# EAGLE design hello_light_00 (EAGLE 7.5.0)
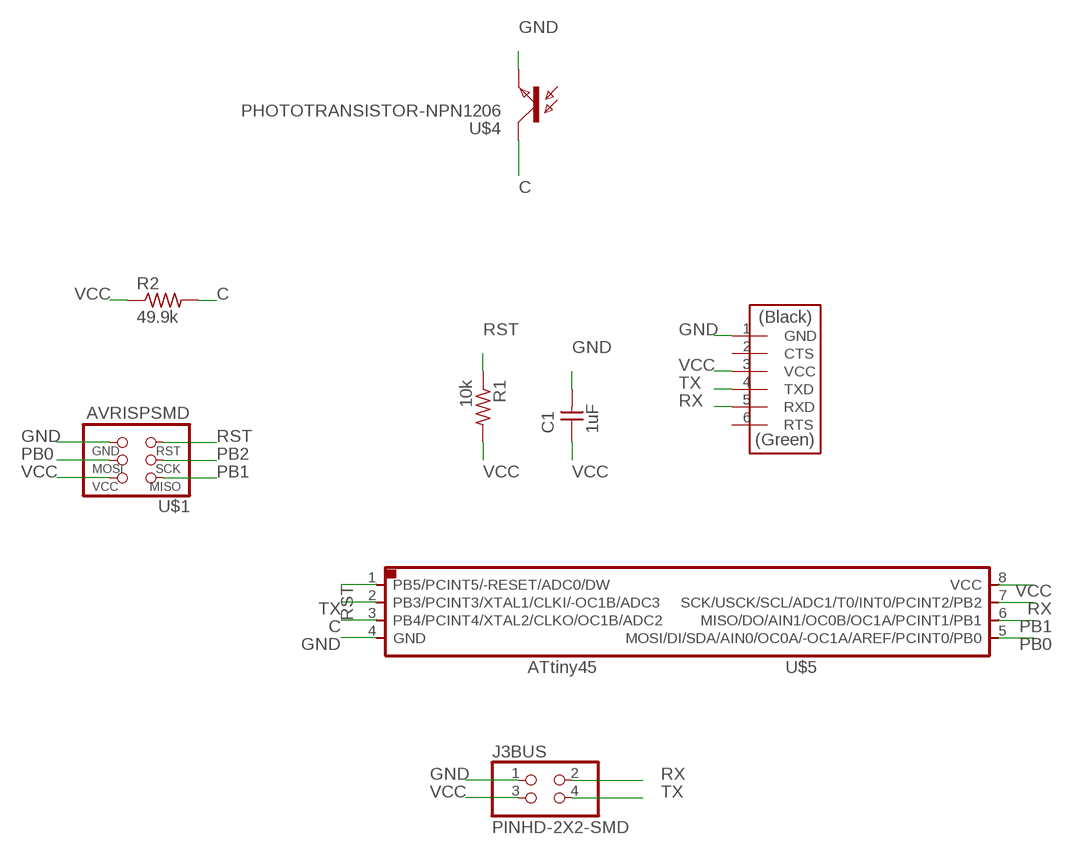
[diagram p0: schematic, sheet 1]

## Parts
C1  1uF  CAP-UNPOLARIZEDFAB  [C1206FAB]
J2FTDI  FTDI-SMD-HEADER  [1X06SMD]
J3BUS  PINHD-2X2-SMD  [2X02SMD]
R1  10k  RES-US1206FAB  [R1206FAB]
R2  49.9k  RES-US1206FAB  [R1206FAB]
U$1  AVRISPSMD  [2X03SMD]
U$4  PHOTOTRANSISTOR-NPN1206  [OP1206]
U$5  ATTINY45SI  [SOIC8]

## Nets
C: R2.2 U$4.COLLECTOR(C) U$5.3(PB4/PCINT4/XTAL2/CLKO/OC1B/ADC2)
GND: C1.2 J2FTDI.1(GND) J3BUS.1 U$1.6(GND) U$4.EMITTER(E) U$5.4(GND)
PB0: U$1.4(MOSI) U$5.5(MOSI/DI/SDA/AIN0/OC0A/-OC1A/AREF/PCINT0/PB0)
PB1: U$1.1(MISO) U$5.6(MISO/DO/AIN1/OC0B/OC1A/PCINT1/PB1)
PB2: U$1.3(SCK)
RST: R1.1 U$1.5(RST) U$5.1(PB5/PCINT5/-RESET/ADC0/DW)
RX: J2FTDI.5(RXD) J3BUS.2 U$5.7(SCK/USCK/SCL/ADC1/T0/INT0/PCINT2/PB2)
TX: J2FTDI.4(TXD) J3BUS.4 U$5.2(PB3/PCINT3/XTAL1/CLKI/-OC1B/ADC3)
VCC: C1.1 J2FTDI.3(VCC) J3BUS.3 R1.2 R2.1 U$1.2(VCC) U$5.8(VCC)
Unconnected: J2FTDI.2(CTS) J2FTDI.6(RTS)

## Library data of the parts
C1 = fab:CAP-UNPOLARIZED
J2FTDI = fab:FTDI-SMD-HEADER
J3BUS = fab:PINHD-2X2-SMD
R1 R2 = fab:RES-US: Resistor (US Symbol)
U$1 = fab:AVRISP
U$4 = fab:PHOTOTRANSISTOR-NPN
U$5 = fab:ATTINY45

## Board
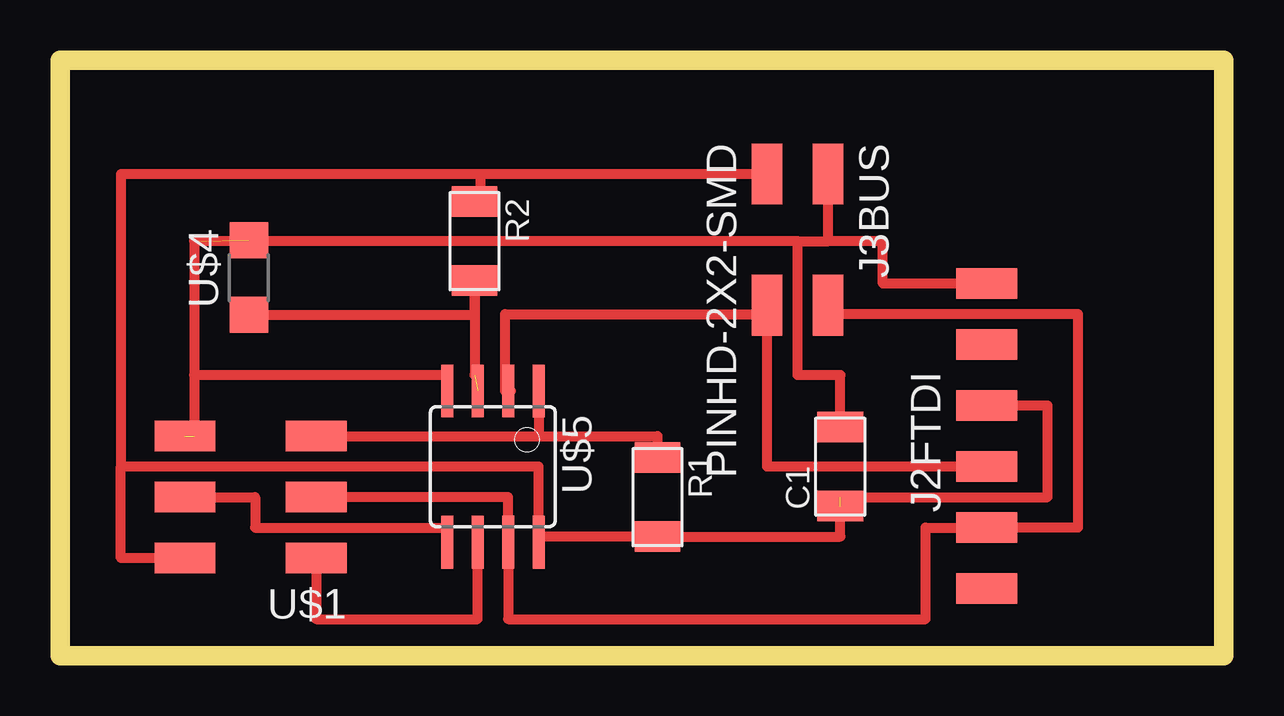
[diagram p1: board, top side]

Size 48.49 x 24.82 mm. Coordinates in mm from the lower left corner, seen from the top.
Outline: 0,0 48.49,0 48.49,24.82 0,24.82 0,0
Copper layers (1*16): Top 0.035mm / dielectric 1.5mm / Bottom 0.035mm
Design rules "default": minimum track width 10mil, minimum drill 24mil, track to track 8mil, track to pad 8mil, pad to pad 8mil, via to via 8mil, smd to smd 8mil, copper to edge 40mil, drill to drill 8mil, minimum pad ring 10mil, minimum via ring 8mil, stop-mask expansion 4mil, vias tented up to drill 0mil, thermal gap 10mil

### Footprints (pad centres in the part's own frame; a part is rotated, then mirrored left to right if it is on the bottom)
C1206FAB = smd 1.27 x 1.905: 1 -1.651,0; 2 1.651,0
1X06SMD = smd 2.54 x 1.27: 1 0,6.35; 2 0,3.81; 3 0,1.27; 4 0,-1.27; 5 0,-3.81; 6 0,-6.35
2X02SMD = smd 2.54 x 1.27: 1 -2.54,1.27; 2 2.92,1.27; 3 -2.54,-1.27; 4 2.92,-1.27
R1206FAB = smd 1.27 x 1.905: 1 -1.651,0; 2 1.651,0
2X03SMD = smd 2.54 x 1.27: 1 -2.54,2.54; 2 2.92,2.54; 3 -2.54,0; 4 2.92,0; 5 -2.54,-2.54; 6 2.92,-2.54
OP1206 = smd 1.5 x 1.6: COLLECTOR -1.55,0; EMITTER 1.55,0
SOIC8 = smd 0.5 x 2.2: 1 -1.905,-3.154; 2 -0.645,-3.154; 3 0.625,-3.154; 4 1.895,-3.154; 5 1.905,3.154; 6 0.635,3.154; 7 -0.635,3.154; 8 -1.905,3.154

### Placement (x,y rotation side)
C1  32.51,7.87 90 top
J2FTDI  38.61,9.14 0 top
J3BUS  30.73,17.53 270 top
R1  24.89,6.6 270 top
R2  17.27,17.27 270 top
U$1  8.13,6.6 180 top
U$4  7.87,15.75 90 top
U$5  18.03,7.87 180 top

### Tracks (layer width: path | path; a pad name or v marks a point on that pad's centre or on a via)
C  (1 unrouted)
  Top 0.406: U$4.COLLECTOR 17.27,14.2 R2.2 17.27,11.68
GND  (2 unrouted)
  Top 0.406: U$5.4 16.14,11.68 5.59,11.68 | 5.59,11.68 5.59,9.14 | 32,17.27 J3BUS.1 | C1.2 32.51,11.68 30.73,11.68 30.73,17.27 | 30.73,17.27 32,17.27 | 30.73,17.27 5.59,17.27 5.59,11.68 | J2FTDI.1 34.29,15.49 34.29,17.27 32,17.27
PB0
  Top 0.406: U$1.4 8.13,6.6 8.13,5.33 16.13,5.33 U$5.5
PB1
  Top 0.406: U$1.1 10.67,1.52 17.4,1.52 U$5.6
RST
  Top 0.406: U$1.5 19.94,9.14 | 19.94,9.14 24.89,9.14 R1.1 | U$5.1 19.94,9.14
RX
  Top 0.406: 10.67,6.6 18.67,6.6 U$5.7 18.67,1.52 36.07,1.52 36.07,5.33 J2FTDI.5 42.42,5.33 42.42,14.22 32.26,14.22 | 32.26,14.22 32,14.22 | J3BUS.2 32.26,14.61 32.26,14.22
TX
  Top 0.406: J2FTDI.4 29.46,7.87 J3BUS.4 29.46,14.22 18.54,14.22 18.54,11.03 U$5.2 18.8,11.03
VCC  (1 unrouted)
  Top 0.406: U$1.2 2.54,4.06 2.54,7.87 | U$5.8 19.94,4.95 | 19.94,4.95 R1.2 32.51,4.95 C1.1 | 19.94,4.95 19.94,7.87 2.54,7.87 | J2FTDI.3 41.15,10.41 41.15,6.6 32.51,6.6 | J3BUS.3 17.53,20.07 | 17.53,20.07 2.54,20.07 2.54,7.87 | R2.1 17.53,18.92 17.53,20.07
